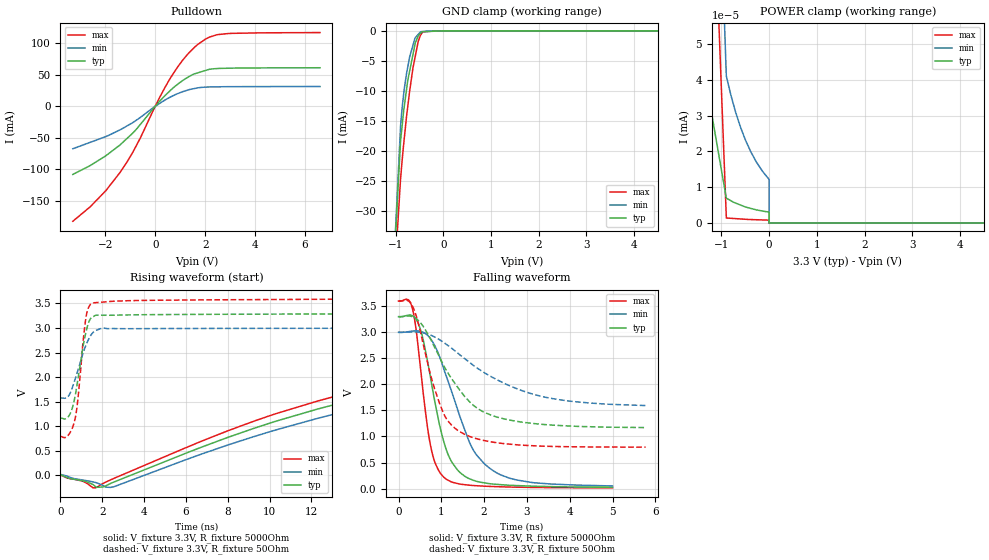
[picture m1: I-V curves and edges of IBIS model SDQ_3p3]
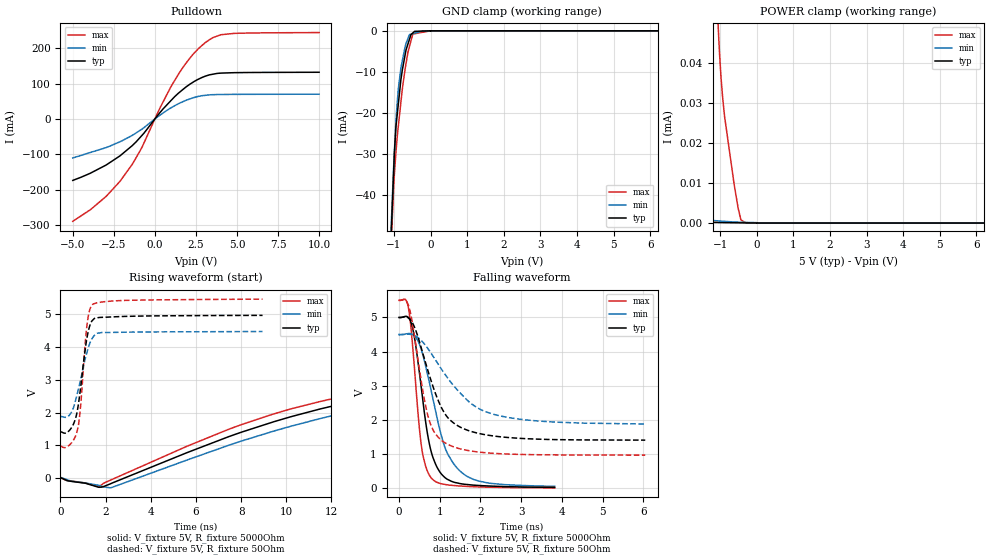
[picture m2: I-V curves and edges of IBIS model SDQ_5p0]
|Texas Instruments Incorporated
| 1.5K Bit Serial EPROM with SDQ Interface
| Marketing part#   Digital Voltage Range   Package-type   #pins
| BQ2024DBZR   2.65V - 5.5V   SOT-23   3
[IBIS Ver]   3.2
[File name]   bq2024.ibs
|SIMDE Ver   V2.2 - 201009 - RHL4 - Build 420
[File Rev]   1.0
[Date]   10/22/2010
[Source]
| Texas Instruments Incorporated.
| Analog-eLab Design Center, HPA
| 12500 TI Blvd
| Dallas, TX -75243
| e-mail: elab_ibis@list.ti.com
| -Model generated from simulations in TISPICE
[Notes]   Revision History:
| Rev 1.0: 10/22/2010
| - Initial version of the model
| - Model generated from simulations in TISPICE
| - Model matched to SPICE simulation
| - Model names with a trailing _3p3 contains the model for
|   3.3V [3.0V and 3.6V]. Model names with trailing _5p0 contains
|   the model for 5.0V [4.5V and 5.5V] operation.
| - C_comp although listed in numerical order of value are
|   obtained from varying PVT conditions. For PVT conditions for
|   each specific value refer the buffer description under
|   respective [Model]. IBIS model user is responsible for using
|   appropriate C_comp to simulate for Signal Integrity.
[Disclaimer]
| This model is designed as an aid for customers of Texas Instruments.
| TI and its licensors and suppliers make no warranties, either expressed
| or implied, with respect to this  model, including the warranties of
| merchantability or fitness for a particular purpose. The model is
| provided solely on an "as is" basis. The entire risk as to its quality
| and performance is with the customer.
[Copyright]
 (C) Copyright 2010 Texas Instruments Incorporated.All rights reserved.
|   BQ2024
[Component]   BQ2024
[Manufacturer]   TI
[Package]   |3 SOT-23 -  DBZ package
|   typ   min   max
R_pkg   0.06396   0.06396   0.06396
L_pkg   1.73579nH   1.73579nH   1.73579nH
C_pkg   0.25854pF   0.25854pF   0.25854pF
[Pin]  signal_name   model_name   R_pin   L_pin   C_pin
1   SDQ   IO   0.06396   1.73579nH  0.25854pF
2   VSS   GND   0.04604   1.35639nH  0.23856pF
3   VSS   GND   0.06894   1.80882nH  0.28151pF
|   Model Selectors
[Model Selector] IO
SDQ_3p3   3.3V digital input
SDQ_5p0   5.0V digital input
| Models and submodels in the file (2): SDQ_3p3 (I/O_open_drain), SDQ_5p0 (I/O_open_drain)
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|   sdq_3p3 Model
[Model]   SDQ_3p3
Model_type   I/O_open_drain
Polarity   Inverting
Enable   Active-Low
Vinl = 0.8
Vinh = 2.2
Vmeas = 1.65
Vref = 3.3
Cref = 15pF
Rref = 5000
|   typ   min   max
|   (nom PVT)   (Fast PVT)   (slow PVT)
C_comp   3.859e-12   3.753e-12   3.984e-12
|ON state : BUFFER OUTPUT TURNED LOW
|C_comp   1.180e-11   1.013e-11   1.489e-11
|OFF state: BUFFER IN HIGH IMPEDANCE
|C_comp   3.859e-12   3.753e-12   3.984e-12
| Where nom  PVT is Nominal Process,  3.3V,  40C
|   Fast PVT is Strong Process,   3.6V,  -20C
|   Slow PVT is Weak Process,   3V,  85C
[Voltage Range]   3.3   3   3.6
|Ambient Temperature   25   70   -20
|Junction Temperature
[Temperature Range]   40   85   -20
[Pullup Reference]   3.3   3   3.6
[Pulldown Reference]   0   0   0
[Power Clamp Reference]   3.3   3   3.6
[GND Clamp Reference]   0   0   0
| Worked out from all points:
|   slope of the pulldown table from 0 to 0.495 V, typ, clamps not added: 23.6 ohm
|   GND clamp passes 1 mA (typ) near -0.54 V on its own axis
|   falling waveform, V_fixture 3.3V, R_fixture 5000Ohm: 20-80 % time 516ps typ, 815ps min, 337ps max; typ from 3.3 V to 0.024 V
|   rising waveform, V_fixture 3.3V, R_fixture 5000Ohm: 20-80 % time 64.4ns typ, 26.9ns min, 63.4ns max; typ from 0.014 V to 3.28 V
|   falling waveform, V_fixture 3.3V, R_fixture 50Ohm: 20-80 % time 1.01ns typ, 1.7ns min, 605ps max; typ from 3.3 V to 1.17 V
|   rising waveform, V_fixture 3.3V, R_fixture 50Ohm: 20-80 % time 503ps typ, 654ps min, 383ps max; typ from 1.17 V to 3.29 V
[Pulldown]
|   Voltage   I(typ)   I(min)   I(max)
-3.3V     -108.2mA   -67.4mA    -182.6mA
-2.599V   -93.98mA   -57.15mA   -159.5mA
-1.98V    -78.65mA   -48.1mA    -134.1mA
-1.404V   -61.16mA   -37.32mA   -104.8mA
-896.4mV  -42.44mA   -25.84mA   -72.95mA
172.8mV   7.838mA    4.427mA    13.78mA
633.6mV   26.24mA    15.24mA    46.41mA
1.246V    44.74mA    25.08mA    80.26mA
1.706V    53.23mA    29.35mA    98.36mA
2.167V    58.84mA    30.77mA    109.9mA
2.934V    60.54mA    31.21mA    115.7mA
6.6V      61.29mA    31.48mA    117.2mA
[GND Clamp]
|   Voltage   I(typ)   I(min)   I(max)
-3.3V     -818.4mA   -761.8mA   -902.3mA
-1.026V   -37.34mA   -36.67mA   -41.21mA
-897mV    -18.22mA   -15.71mA   -24.52mA
-864mV    -15.71mA   -12.68mA   -21.49mA
-819mV    -12.49mA   -9.597mA   -17.78mA
-745.8mV  -8.168mA   -5.962mA   -12.51mA
-637.2mV  -3.885mA   -2.376mA   -6.147mA
-587.4mV  -1.968mA   -1.121mA   -4.142mA
-529.2mV  -874.1uA   -607.8uA   -1.798mA
-477mV    -392.9uA   -147.6uA   -680.8uA
-133.2mV  -45.67uA   -1.141uA   -13.99nA
6.6V      0A         0A         0A
[POWER Clamp]
|   Voltage   I(typ)   I(min)   I(max)
-3.3V     4.424uA    1.524uA    229uA
-2.315V   115.8nA    588.2nA    493.4nA
-897.6mV  6.957nA    41.25nA    1.82nA
-896.4mV  6.947nA    40.99nA    1.404nA
-804mV    6.248nA    35.82nA    1.323nA
-708mV    5.607nA    31.2nA     1.239nA
-606mV    5.063nA    27nA       1.149nA
-501mV    4.504nA    23.33nA    1.057nA
-267mV    3.675nA    17.03nA    924.1pA
-33.83fV  3.054nA    12.18nA    814.1pA
0V        0A         0A         0A
6.6V      0A         0A         0A
[Ramp]
R_load = 5000
|   typ   min   max
dV/dt_r   1.96196/6.35417e-08   1.77785/2.67709e-08   2.14505/6.08055e-08
dV/dt_f   1.97155/5.19489e-10   1.78703/8.34251e-10   2.15474/3.37364e-10
[Falling Waveform]
V_fixture = 3.3V
V_fixture_min = 3V
V_fixture_max = 3.6V
R_fixture = 5000Ohm
|   Time   V(typ)   V(min)   V(max)
0s        3.3V       3V         3.6V
300ps     3.327V     3.02V      3.524V
475ps     3.144V     3.024V     2.594V
750ps     2.122V     2.875V     818.5mV
1.075ns   852.5mV    2.252V     205.2mV
1.375ns   361.2mV    1.531V     97.04mV
1.7ns     174.9mV    811.9mV    61.23mV
2.2ns     86.96mV    349.9mV    39.15mV
3.125ns   46.18mV    115.4mV    21.6mV
5ns       24.49mV    50.11mV    13.37mV
[Rising Waveform]
V_fixture = 3.3V
V_fixture_min = 3V
V_fixture_max = 3.6V
R_fixture = 5000Ohm
|   Time   V(typ)   V(min)   V(max)
0s        14.07mV    21.56mV    8.758mV
1.55ns    -183.1mV   -129.8mV   -249.2mV
2.525ns   -138.9mV   -231.8mV   -65.1mV
9.95ns    1.056V     882mV      1.207V
15.6ns    1.688V     1.489V     1.856V
27.25ns   2.331V     2.18V      2.405V
49.85ns   2.55V      2.563V     2.718V
146.3ns   2.974V     2.649V     3.316V
305.5ns   3.237V     2.902V     3.55V
800ns     3.284V     2.985V     3.584V
[Falling Waveform]
V_fixture = 3.3V
V_fixture_min = 3V
V_fixture_max = 3.6V
R_fixture = 50Ohm
|   Time   V(typ)   V(min)   V(max)
0s        3.3V       3V         3.6V
325ps     3.299V     3.008V     3.506V
575ps     3.116V     2.99V      2.778V
975ps     2.497V     2.849V     1.602V
1.125ns   2.26V      2.765V     1.333V
1.425ns   1.896V     2.572V     1.095V
1.95ns    1.486V     2.253V     931mV
2.575ns   1.318V     1.982V     853.7mV
3.75ns    1.211V     1.707V     806.1mV
5.775ns   1.171V     1.594V     794.8mV
[Rising Waveform]
V_fixture = 3.3V
V_fixture_min = 3V
V_fixture_max = 3.6V
R_fixture = 50Ohm
|   Time   V(typ)   V(min)   V(max)
0s        1.165V     1.575V     791.2mV
400ps     1.211V     1.626V     835.2mV
700ps     1.612V     1.956V     1.154V
825ps     1.932V     2.125V     1.516V
1.05ns    2.553V     2.445V     2.586V
1.2ns     2.878V     2.629V     3.16V
1.3ns     3.051V     2.729V     3.37V
1.475ns   3.21V      2.866V     3.496V
2.075ns   3.259V     2.996V     3.528V
14.02ns   3.287V     2.995V     3.587V
|   sdq_5p0 Model
[Model]   SDQ_5p0
Model_type   I/O_open_drain
Polarity   Inverting
Enable   Active-Low
Vinl = 0.8
Vinh = 2.2
Vmeas = 2.5
Vref = 5.0
Cref = 15pF
Rref = 5000
|   typ   min   max
|   (nom PVT)   (Fast PVT)   (slow PVT)
C_comp   3.522e-12   3.415e-12   3.660e-12
|ON state : BUFFER OUTPUT TURNED LOW
|C_comp   1.127e-11   9.859e-12   1.424e-11
|OFF state: BUFFER IN HIGH IMPEDANCE
|C_comp   3.522e-12   3.415e-12   3.660e-12
| Where nom  PVT is Nominal Process,  5V,  40C
|   Fast PVT is Strong Process,   5.5V,  -20C
|   Slow PVT is Weak Process,   4.5V,  85C
[Voltage Range]   5   4.5   5.5
|Ambient Temperature   25   70   -20
|Junction Temperature
[Temperature Range]   40   85   -20
[Pullup Reference]   5   4.5   5.5
[Pulldown Reference]   0   0   0
[Power Clamp Reference]   5   4.5   5.5
[GND Clamp Reference]   0   0   0
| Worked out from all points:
|   slope of the pulldown table from 0 to 0.75 V, typ, clamps not added: 18.4 ohm
|   GND clamp passes 1 mA (typ) near -0.54 V on its own axis
|   falling waveform, V_fixture 5V, R_fixture 5000Ohm: 20-80 % time 371ps typ, 576ps min, 250ps max; typ from 5 V to 0.032 V
|   rising waveform, V_fixture 5V, R_fixture 5000Ohm: 20-80 % time 33.7ns typ, 36.4ns min, 32.7ns max; typ from 0.017 V to 4.96 V
|   falling waveform, V_fixture 5V, R_fixture 50Ohm: 20-80 % time 654ps typ, 1.09ns min, 413ps max; typ from 5 V to 1.41 V
|   rising waveform, V_fixture 5V, R_fixture 50Ohm: 20-80 % time 404ps typ, 543ps min, 313ps max; typ from 1.41 V to 4.97 V
[Pulldown]
|   Voltage   I(typ)   I(min)   I(max)
-5V       -174mA     -110.6mA   -289.8mA
-3.921V   -153.5mA   -94.89mA   -256.8mA
-2.98V    -130.8mA   -81.22mA   -219.7mA
-2.123V   -104.5mA   -64.52mA   -176.6mA
-907.5mV  -52.82mA   -32.56mA   -90.9mA
335.5mV   19.33mA    11.47mA    33.48mA
1.468V    74.22mA    43.81mA    129.1mA
2.272V    102.4mA    58.91mA    180mA
3.08V     121.2mA    66.87mA    216.4mA
4.01V     129.7mA    69.17mA    238.2mA
4.84V     130.9mA    69.5mA     242.1mA
10V       132.1mA    69.99mA    244.5mA
[GND Clamp]
|   Voltage   I(typ)   I(min)   I(max)
-5V       -1.545A    -1.437A    -1.701A
-1.103V   -55.62mA   -53.52mA   -59.61mA
-1.062V   -46.34mA   -44.56mA   -48.9mA
-990mV    -30.16mA   -29.57mA   -35.1mA
-945mV    -23.3mA    -21.89mA   -29.48mA
-882mV    -17.95mA   -14.23mA   -23.32mA
-810mV    -11.84mA   -9.074mA   -17.38mA
-670mV    -4.651mA   -3.075mA   -7.964mA
-616mV    -3.158mA   -1.834mA   -5.117mA
-484mV    -512.6uA   -689.5uA   -783.2uA
-435mV    -122.6uA   -569.5uA   -703.9uA
10V       0A         0A         0A
[POWER Clamp]
|   Voltage   I(typ)   I(min)   I(max)
-5V       326.3uA    238.7uA    444.2uA
-3.276V   238.1uA    48.82uA    341.3uA
-3.123V   230.3uA    33.05uA    332.2uA
-2.556V   201.3uA    5.801uA    298.3uA
-2.245V   66.96uA    3.566uA    279.8uA
-1.86V    17.39uA    2.372uA    256.9uA
-1.375V   261.2nA    868.8nA    209.4uA
-1.05V    138.2nA    539.2nA    48.89uA
-907.5mV  107.2nA    444.5nA    29.21uA
-616mV    69.22nA    270.3nA    9.648uA
-291.5mV  38.74nA    167.2nA    13.07nA
10V       0A         0A         0A
[Ramp]
R_load = 5000
|   typ   min   max
dV/dt_r   2.97843/3.42983e-08   2.67461/3.74478e-08   3.28229/3.30138e-08
dV/dt_f   2.98993/3.73272e-10   2.68485/5.90974e-10   3.29359/2.50508e-10
[Falling Waveform]
V_fixture = 5V
V_fixture_min = 4.5V
V_fixture_max = 5.5V
R_fixture = 5000Ohm
|   Time   V(typ)   V(min)   V(max)
0s        5V         4.499V     5.5V
200ps     5.026V     4.524V     5.441V
325ps     4.745V     4.509V     4.323V
550ps     2.943V     4.057V     1.26V
675ps     1.793V     3.477V     583.6mV
800ps     1.042V     2.816V     297.9mV
1.125ns   324.1mV    1.213V     119.6mV
1.55ns    132.7mV    458.6mV    68.89mV
2.225ns   71.55mV    154.6mV    36.52mV
3.825ns   32.13mV    61.88mV    18.06mV
[Rising Waveform]
V_fixture = 5V
V_fixture_min = 4.5V
V_fixture_max = 5.5V
R_fixture = 5000Ohm
|   Time   V(typ)   V(min)   V(max)
0s        16.67mV    24.73mV    10.65mV
2.225ns   -169.2mV   -292.9mV   -57.74mV
7.825ns   1.358V     1.09V      1.587V
12.2ns    2.227V     1.934V     2.448V
22.78ns   3.177V     3.002V     3.419V
40.28ns   3.971V     3.514V     4.44V
71.15ns   4.609V     3.902V     5.128V
112.7ns   4.69V      3.962V     5.281V
192.3ns   4.427V     4.077V     4.848V
499.6ns   4.955V     4.457V     5.462V
[Falling Waveform]
V_fixture = 5V
V_fixture_min = 4.5V
V_fixture_max = 5.5V
R_fixture = 50Ohm
|   Time   V(typ)   V(min)   V(max)
0s        5V         4.5V       5.5V
175ps     5.015V     4.51V      5.491V
275ps     4.944V     4.507V     5.179V
600ps     3.896V     4.26V      2.761V
750ps     3.299V     4.025V     1.969V
875ps     2.849V     3.8V       1.634V
1.125ns   2.194V     3.35V      1.34V
1.75ns    1.676V     2.505V     1.099V
2.375ns   1.527V     2.152V     1.024V
6.05ns    1.414V     1.885V     974.5mV
[Rising Waveform]
V_fixture = 5V
V_fixture_min = 4.5V
V_fixture_max = 5.5V
R_fixture = 50Ohm
|   Time   V(typ)   V(min)   V(max)
0s        1.409V     1.879V     971.8mV
425ps     1.48V      1.948V     1.029V
750ps     2.067V     2.587V     1.47V
875ps     2.662V     2.956V     2.072V
1.075ns   3.815V     3.585V     3.93V
1.175ns   4.288V     3.846V     4.669V
1.3ns     4.655V     4.115V     5.15V
1.45ns    4.84V      4.313V     5.316V
1.875ns   4.911V     4.448V     5.381V
8.95ns    4.97V      4.476V     5.466V
